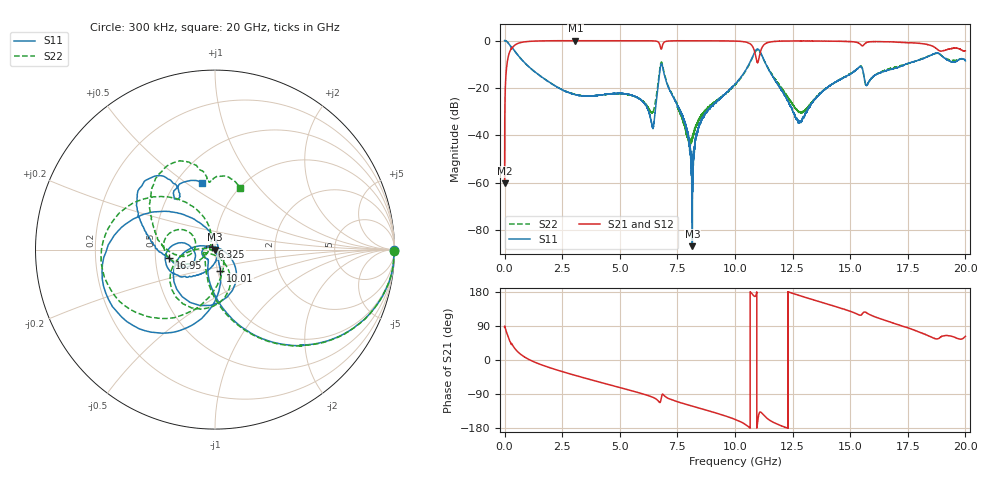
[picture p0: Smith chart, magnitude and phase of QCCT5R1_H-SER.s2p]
!{QCCT5R1}
!Johanson Technology Inc.
!www.johansontechnology.com
!Test Board Conditions:
!Substrate Type  RO4350B
!Substrate Thickness  20 mil
!Substrate Dk  3.66
!TL Type: GCPW
!TL Trace Width  34 mil
!TL Gap  10 mil
!Electrode orientation  Horizontal
!DUT TOPOLOGY	SERIES
!Mounting Pad LxW  26x52 mil
# MHz S  dB  R 50
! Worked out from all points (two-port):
!   20001 points, 300 kHz to 20 GHz, reference 50 ohm
!   highest |S21| = -0.05 dB at 3.074 GHz (marker M1); lowest = -60.2 dB at 300 kHz (marker M2)
!   |S21| within 3 dB of the highest: 332 MHz to 6.77 GHz (6.438 GHz wide, 181 % of centre); 11.17 GHz to 18.7 GHz (7.527 GHz wide, 50.4 % of centre)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
!   lowest |S11| = -86.8 dB at 8.148 GHz (marker M3), VSWR 1.00, Z = 50 + j0.00457 ohm
!   |S11| at or under -10 dB: 935.6 MHz to 6.79 GHz (5.855 GHz wide, 152 % of centre); 6.83 GHz to 10.61 GHz (3.778 GHz wide, 43.3 % of centre); 11.34 GHz to 17.41 GHz (6.066 GHz wide, 42.2 % of centre)
!   |S22| runs from -45.1 to 0.0 dB; largest |S21 - S12| = 0.017
!   S11 on the Smith chart (normalised r, x): 300 kHz: open; 6.325 GHz: 0.97, +0.03; 10.01 GHz: 1.03, -0.25; 16.95 GHz: 0.59, -0.06; 20 GHz: 0.67, +0.57
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0.3  -0.02 -0.1  -60.24 86.4  -60.21 91.5  -0.02 -0.3
113.298  -0.56 -21.9  -9.23 67.8  -9.22 67.7  -0.55 -22.0
323.295  -2.92 -48.4  -3.17 41.1  -3.16 41.1  -2.93 -48.6
1095.284  -11.43 -88.5  -0.34 0.2  -0.35 0.3  -11.46 -90.6
3074.254  -22.86 -121.1  -0.05 -40.8  -0.05 -40.7  -22.74 -139.5
3334.25  -23.32 -124.3  -0.06 -45.2  -0.07 -45.2  -23.24 -145.8
5531.217  -23.16 -176.1  -0.09 -81.4  -0.09 -81.4  -23.21 -166.0
6325.205  -32.64 132.5  -0.12 -95.9  -0.11 -95.8  -30.05 -131.2
6667.2  -18.84 -31.7  -0.61 -107.8  -0.63 -107.8  -17.59 -56.2
6864.197  -11.31 -148.6  -1.74 -90.2  -1.73 -90.0  -10.83 -150.3
7825.183  -34.63 140.5  -0.10 -116.1  -0.10 -116.1  -36.52 -168.9
8148.178  -86.78 94.0  -0.10 -121.8  -0.10 -121.8  -41.08 -63.4
8621.171  -32.37 -59.7  -0.10 -130.0  -0.10 -130.0  -30.54 -34.5
10000.15  -18.43 -76.0  -0.23 -156.7  -0.24 -156.6  -18.77 -66.7
10006.15  -18.36 -76.1  -0.23 -156.8  -0.24 -156.7  -18.69 -67.1
10993.14  -3.68 -160.3  -9.27 -158.6  -9.18 -158.6  -3.92 -175.7
11277.13  -8.65 145.0  -1.65 -147.5  -1.59 -147.7  -8.66 128.6
12720.11  -33.66 28.4  -0.18 171.6  -0.19 171.5  -29.72 139.1
13334.1  -26.45 -74.6  -0.19 160.1  -0.18 160.1  -26.10 -155.2
16667.05  -12.45 -162.0  -0.52 101.5  -0.64 101.5  -12.02 -176.8
16945.05  -11.68 -169.2  -0.63 95.8  -0.68 95.6  -11.24 179.2
20000  -8.55 100.9  -4.33 62.4  -4.37 62.5  -8.73 67.4
